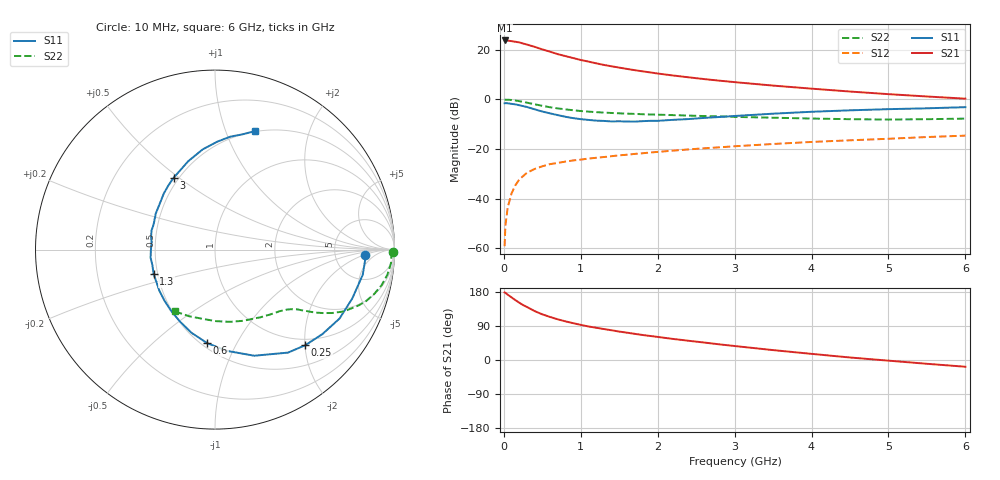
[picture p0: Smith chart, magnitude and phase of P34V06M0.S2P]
! SIEMENS Small Signal Semiconductors
! BFP181
! Si NPN RF Bipolar Junction Transistor in SOT143
! VCE = 4 V  IC = 6 mA
! Common Emitter S-Parameters:  March  1996
# GHz  S  MA  R  50
!  f  S11  S21  S12  S22
! GHz  MAG  ANG  MAG  ANG  MAG  ANG  MAG  ANG
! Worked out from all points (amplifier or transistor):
!   36 points, 10 MHz to 6 GHz, reference 50 ohm
!   highest |S21| = 23.7 dB at 10 MHz (marker M1)
!   |S21| within 3 dB of that: start of sweep to 442.2 MHz
!   unconditionally stable (mu >= 1): 1.58 GHz to end of sweep
!   at 250 MHz: K = 0.24, MSG = 26.7 dB, |S12| = -30.9 dB
!   at 1.4 GHz: K = 0.95, MSG = 18.1 dB, |S12| = -22.9 dB
!   at 6 GHz: K = 1.03, MAG = 6.4 dB, |S12| = -14.6 dB
!   S11 on the Smith chart (normalised r, x): 10 MHz: 11, -2; 250 MHz: 0.87, -2.00; 600 MHz: 0.53, -0.77; 1.3 GHz: 0.48, -0.15; 3 GHz: 0.47, +0.48; 6 GHz: 0.49, +1.27
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0.01  0.8335 -2.0  15.39 178.3  0.0011 83.9  0.9891 -0.7
0.02  0.8384 -4.1  15.27 177.3  0.0028 92.1  0.9835 -1.6
0.05  0.835 -9.7  15.31 172.4  0.0066 90.1  0.9842 -4.2
0.15  0.793 -29.0  14.49 158.0  0.0186 74.0  0.949 -12.1
0.2  0.7614 -38.2  14.07 151.3  0.0242 70.2  0.9206 -15.6
0.25  0.7325 -46.7  13.36 145.0  0.0284 66.6  0.8895 -18.8
0.3  0.7033 -54.7  12.73 139.9  0.0331 62.8  0.859 -21.2
0.4  0.6304 -69.7  11.46 129.1  0.0396 57.3  0.797 -25.6
0.5  0.5685 -83.2  10.17 120.5  0.0448 52.8  0.7407 -28.5
0.6  0.5231 -94.8  9.151 113.6  0.0495 49.8  0.6944 -30.6
0.7  0.4816 -105.8  8.161 107.4  0.0524 47.4  0.6579 -32.2
0.8  0.4459 -116.0  7.459 102.0  0.0557 46.1  0.6289 -33.3
0.9  0.419 -126.0  6.81 97.2  0.0588 44.7  0.604 -34.3
1.1  0.3853 -143.7  5.775 88.5  0.0642 43.3  0.5663 -36.0
1.3  0.3678 -158.5  4.946 81.7  0.0688 42.4  0.5418 -37.8
1.7  0.3556 173.9  3.877 69.1  0.0796 41.3  0.5094 -41.8
2.2  0.3867 148.5  3.026 55.6  0.0926 39.9  0.4814 -47.7
3  0.4623 119.8  2.226 36.9  0.1134 35.9  0.4436 -59.5
3.5  0.5148 106.8  1.895 26.1  0.1262 33.0  0.4269 -68.3
4.5  0.6015 88.8  1.438 6.6  0.1497 26.5  0.3987 -89.2
5.5  0.6606 76.5  1.143 -10.0  0.1741 20.2  0.3985 -111.4
6  0.6965 71.4  1.033 -17.8  0.1858 16.6  0.4098 -122.7
